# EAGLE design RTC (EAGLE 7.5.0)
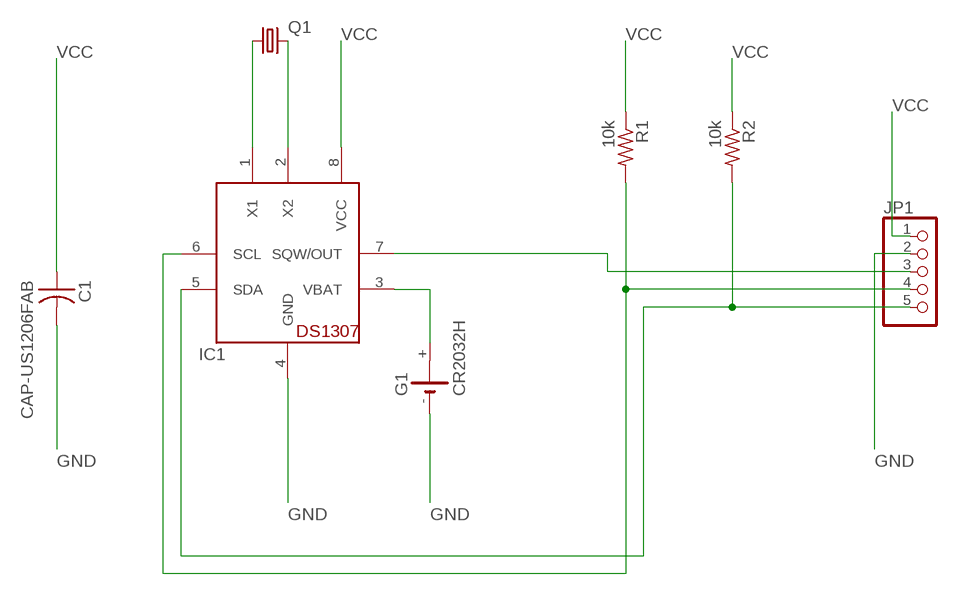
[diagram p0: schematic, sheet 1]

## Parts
C1  CAP-US1206FAB  [C1206FAB]
G1  CR2032H  [CR2032H]
IC1  DS1307  [DIL08]
JP1  PINHD-1X5  [1X05]
Q1  CRYSTALTC38H  [TC38H]
R1  10k  RES-US1206FAB  [R1206FAB]
R2  10k  RES-US1206FAB  [R1206FAB]

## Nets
GND: C1.2 G1.- IC1.4(GND) JP1.2
N$1: IC1.1(X1) Q1.1
N$2: IC1.2(X2) Q1.2
N$3: G1.+ IC1.3(VBAT)
N$11: IC1.7(SQW/OUT) JP1.3
N$12: IC1.6(SCL) JP1.4 R1.2
N$13: IC1.5(SDA) JP1.5 R2.2
VCC: C1.1 IC1.8(VCC) JP1.1 R1.1 R2.1
Unconnected: G1.+@1(+)

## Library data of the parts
C1 = fab:CAP-US
G1 = battery:CR2032H: LI BATTERY Varta
IC1 = adafruit:DS1307: DS1307 Real time clock (RTC) with battery backup ability. Talk to it via i2c
JP1 = pinhead:PINHD-1X5: PIN HEADER
Q1 = adafruit:CRYSTAL: CRYSTAL; OC_FARNELL: unknown; OC_NEWARK: unknown
R1 R2 = fab:RES-US: Resistor (US Symbol)

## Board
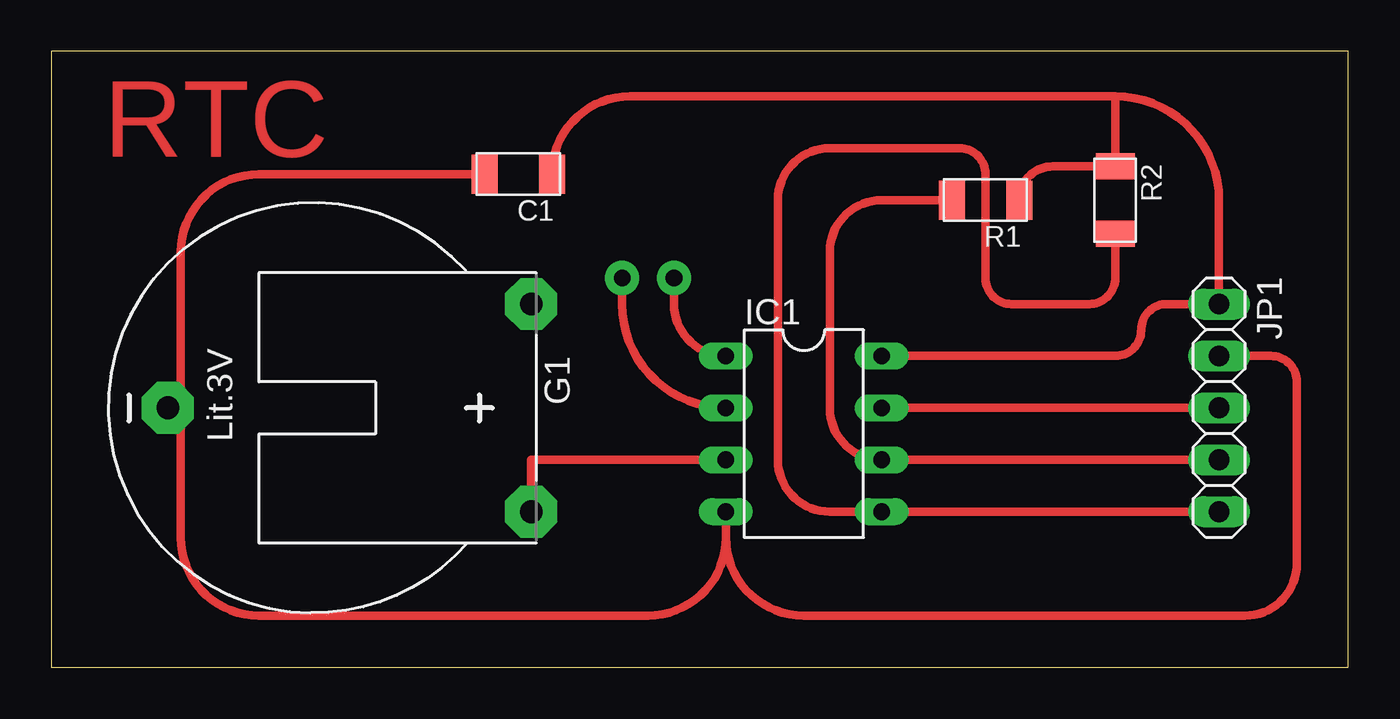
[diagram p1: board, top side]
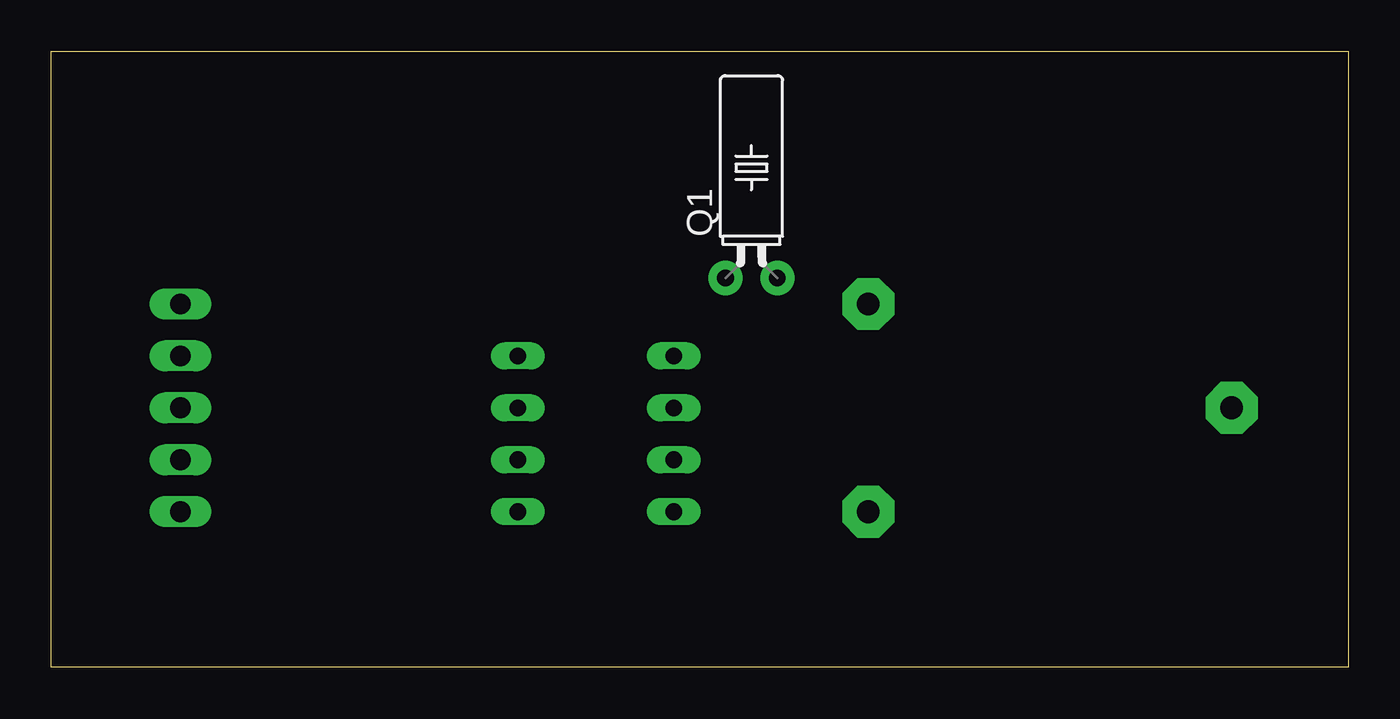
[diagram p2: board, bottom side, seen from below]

Size 63.48 x 30.15 mm. Coordinates in mm from the lower left corner, seen from the top.
Outline: 0,0 63.48,0 63.48,30.15 0,30.15 0,0
Copper layers (1*16): Top 0.035mm / dielectric 1.5mm / Bottom 0.035mm
Design rules "default": minimum track width 10mil, minimum drill 24mil, track to track 8mil, track to pad 8mil, pad to pad 8mil, via to via 8mil, smd to smd 8mil, copper to edge 40mil, drill to drill 8mil, minimum pad ring 10mil, minimum via ring 8mil, stop-mask expansion 4mil, vias tented up to drill 0mil, thermal gap 10mil

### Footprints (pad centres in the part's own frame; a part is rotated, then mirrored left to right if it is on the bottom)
C1206FAB = smd 1.27 x 1.905: 1 -1.651,0; 2 1.651,0
CR2032H = drill 1.118 pad 2.54 octagon: + 5.08,10.795; +@1 -5.08,10.795; - 0,-6.985
DIL08 = drill 0.813 long: 1 -3.81,-3.81; 2 -1.27,-3.81; 3 1.27,-3.81; 4 3.81,-3.81; 5 3.81,3.81; 6 1.27,3.81; 7 -1.27,3.81; 8 -3.81,3.81
1X05 = drill 1.016 long: 1 -5.08,0; 2 -2.54,0; 3 0,0; 4 2.54,0; 5 5.08,0
TC38H = drill 0.813 pad 1.676: 1 -1.27,0; 2 1.27,0
R1206FAB = smd 1.27 x 1.905: 1 -1.651,0; 2 1.651,0

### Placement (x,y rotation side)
C1  22.86,24.13 180 top
G1  12.7,12.7 270 top
IC1  36.83,11.43 270 top
JP1  57.15,12.7 270 top
Q1  29.21,19.05 0 bottom
R1  45.72,22.86 180 top
R2  52.07,22.86 270 top

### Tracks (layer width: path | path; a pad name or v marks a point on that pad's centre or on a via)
GND
  Top 0.406: IC1.4 33.02,6.35 | 33.02,6.35 arc-90 29.21,2.54 10.16,2.54 arc-90 6.35,6.35 6.35,12.06 arc90 G1.- arc90 6.35,13.34 6.35,20.32 arc-90 10.16,24.13 C1.2 | JP1.2 59.69,15.24 arc-90 60.96,13.97 60.96,5.08 arc-90 58.42,2.54 36.83,2.54 arc-90 33.02,6.35
N$1
  Top 0.406: Q1.1 30.48,17.78 arc90 IC1.1
N$2
  Top 0.406: Q1.2 27.94,17.78 arc90 IC1.2
N$3
  Top 0.406: IC1.3 23.5,10.16 G1.+
N$11
  Top 0.406: JP1.3 IC1.7
N$12
  Top 0.406: JP1.4 IC1.6 arc-90 38.1,12.7 38.1,20.32 arc-90 40.64,22.86 R1.2
N$13
  Top 0.406: JP1.5 IC1.5 38.1,7.62 arc-90 35.56,10.16 35.56,22.86 arc-90 38.1,25.4 44.45,25.4 arc-90 45.72,24.13 45.72,19.05 arc90 46.99,17.78 50.8,17.78 arc90 52.07,19.05 R2.2
VCC
  Top 0.406: 52.07,27.94 arc-90 57.15,22.86 JP1.1 54.61,17.78 arc90 53.34,16.51 arc-90 52.07,15.24 IC1.8 | 52.07,27.94 28.32,27.94 arc90 C1.1 | 52.07,27.94 R2.1 49.02,24.51 arc90 R1.1

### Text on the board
Top: RTC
